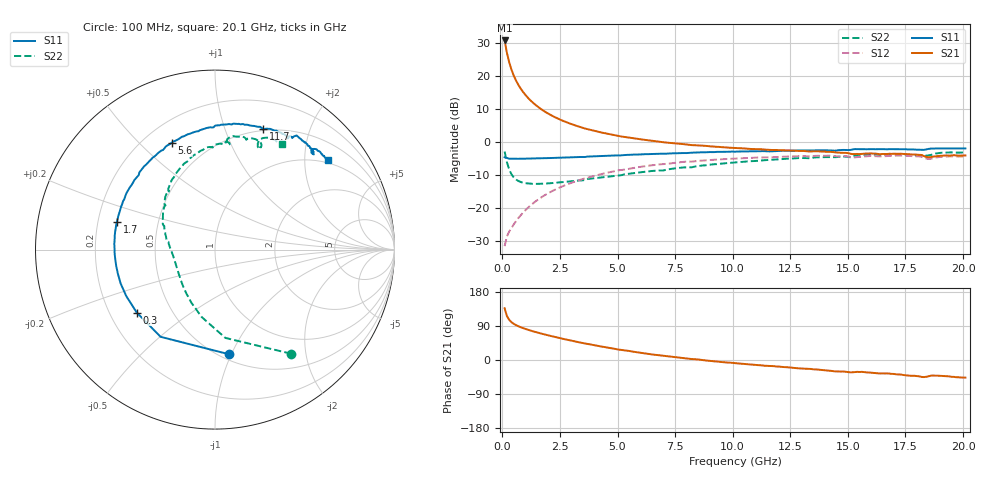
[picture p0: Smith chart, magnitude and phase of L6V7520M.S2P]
!  Infineon Technologies AG
! BFR380L3 , PF131585-7, No.6, Th 09.10.01, soldered on pcb-board, measured with PP GSG850
!  Vce=0.75 V,  Ic=20.0 mA
! Common Emitter S-Parameters:  15. November 2001
#  GHz  S  MA  R  50
! f  S11  S21  S12  S22
! GHz  Mag  Ang  Mag  Ang  Mag  Ang  Mag  Ang
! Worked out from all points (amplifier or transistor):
!   201 points, 100 MHz to 20.1 GHz, reference 50 ohm
!   highest |S21| = 30.8 dB at 100 MHz (marker M1)
!   |S21| within 3 dB of that: start of sweep to 180.2 MHz
!   unconditionally stable (mu >= 1): 1.261 GHz to 4.996 GHz; 5.005 GHz to 5.246 GHz; 18.37 GHz to 18.51 GHz
!   at 3.4 GHz: K = 1.03, MAG = 7.0 dB, |S12| = -11.4 dB
!   at 10.1 GHz: K = 0.98, MSG = 1.6 dB, |S12| = -5.0 dB
!   at 20.1 GHz: K = 0.99, MSG = 0.1 dB, |S12| = -4.3 dB
!   S11 on the Smith chart (normalised r, x): 100 MHz: 0.55, -0.98; 300 MHz: 0.31, -0.32; 1.7 GHz: 0.28, +0.13; 5.6 GHz: 0.31, +0.63; 11.7 GHz: 0.48, +1.37; 20.1 GHz: 0.93, +2.58
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0.1  0.5879 -82.5  34.67 136.4  0.02639 58.5  0.719 -53.8
0.2  0.5727 -121.9  22.54 116.0  0.0371 51.0  0.4953 -83.3
0.3  0.5596 -141.2  16.15 106.0  0.04408 51.0  0.3827 -101.2
0.4  0.5582 -152.5  12.46 99.8  0.05007 52.7  0.3238 -114.0
0.5  0.5586 -160.3  10.11 95.3  0.05671 55.3  0.2903 -123.7
0.6  0.5576 -166.0  8.497 91.9  0.06357 57.1  0.2699 -131.3
0.7  0.5578 -170.6  7.335 89.0  0.07064 58.6  0.2568 -137.6
0.8  0.5583 -174.4  6.444 86.4  0.07778 60.0  0.2479 -142.7
1  0.5597 179.5  5.196 82.0  0.09266 61.4  0.238 -150.8
1.2  0.5619 174.4  4.359 78.1  0.1076 62.2  0.234 -156.8
1.4  0.565 170.1  3.759 74.6  0.1229 62.3  0.2324 -161.7
1.7  0.5678 164.1  3.126 69.6  0.1457 61.7  0.2333 -167.6
2.1  0.5728 157.1  2.57 63.5  0.1758 60.3  0.2379 -173.6
2.5  0.5784 150.8  2.193 57.7  0.2052 58.2  0.2438 -178.9
3.5  0.5938 136.4  1.639 44.7  0.2761 51.7  0.263 170.5
5.6  0.6423 112.1  1.155 22.7  0.3995 36.7  0.3339 150.5
6.8  0.6644 100.3  1.013 12.3  0.4576 28.1  0.3707 139.0
10.1  0.7145 76.6  0.8107 -8.3  0.5611 6.9  0.4909 113.8
11.7  0.725 68.1  0.7582 -16.0  0.5883 -2.4  0.5409 102.1
13.5  0.7473 59.5  0.724 -24.5  0.6129 -12.6  0.5795 90.6
16.8  0.7803 47.7  0.6649 -35.8  0.615 -27.4  0.6503 72.4
20.1  0.8007 38.3  0.6264 -46.6  0.6078 -40.3  0.6967 57.8
